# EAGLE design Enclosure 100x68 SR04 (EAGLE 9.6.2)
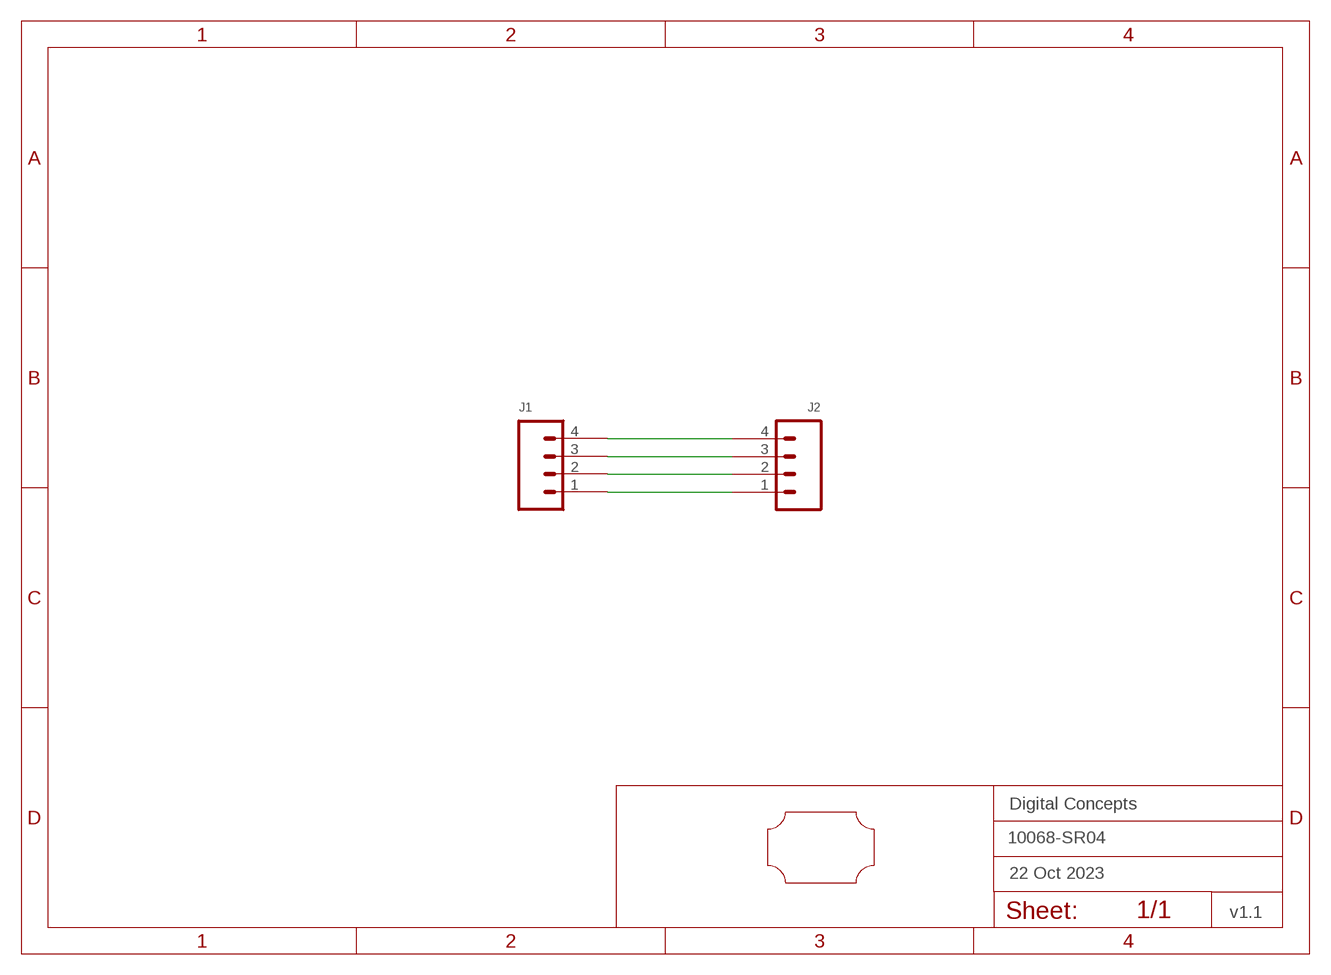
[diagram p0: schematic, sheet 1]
FRAME2 (FRAME_A5L-LOC): DATE: 22 Oct 2023; OWNER: Digital Concepts; TITLE: 10068-SR04; VERSION: v1.1

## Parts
J1  HEADER-1X4-GENERIC  [CONN_04-GENERIC]
J2  JST-XH2.54-4-HORIZONTAL  [JST-XH2.4-4-HORIZONTAL]
U$1  PROTO-34X22-SR04  [PROTO-34X22-SR04]

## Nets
N$1: J1.4 J2.4
N$2: J1.3 J2.3
N$3: J1.2 J2.2
N$4: J1.1 J2.1

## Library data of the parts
J1 = digitalconcepts:HEADER-1X4-GENERIC: Single Row 4-Pin Header
J2 = digitalconcepts:JST-XH2.54-4-HORIZONTAL: XH2.54 4P Horizontal Connector
U$1 = digitalconcepts:PROTO-34X22-SR04: 34 x 22 Prototyping board to fit an 100 x 68 enclosure—AJ-SR04M support

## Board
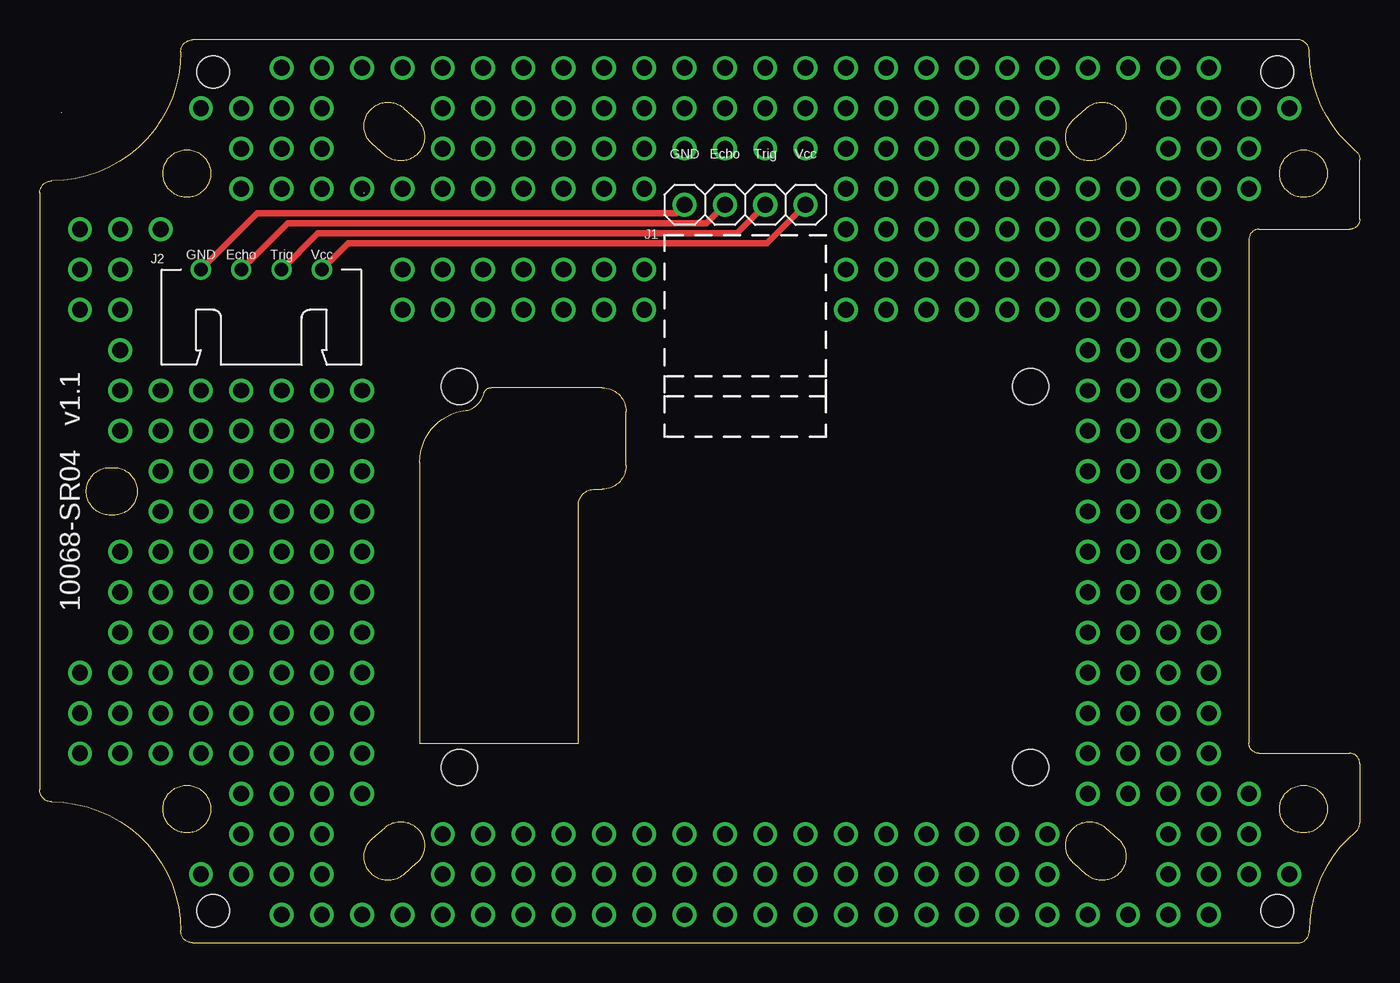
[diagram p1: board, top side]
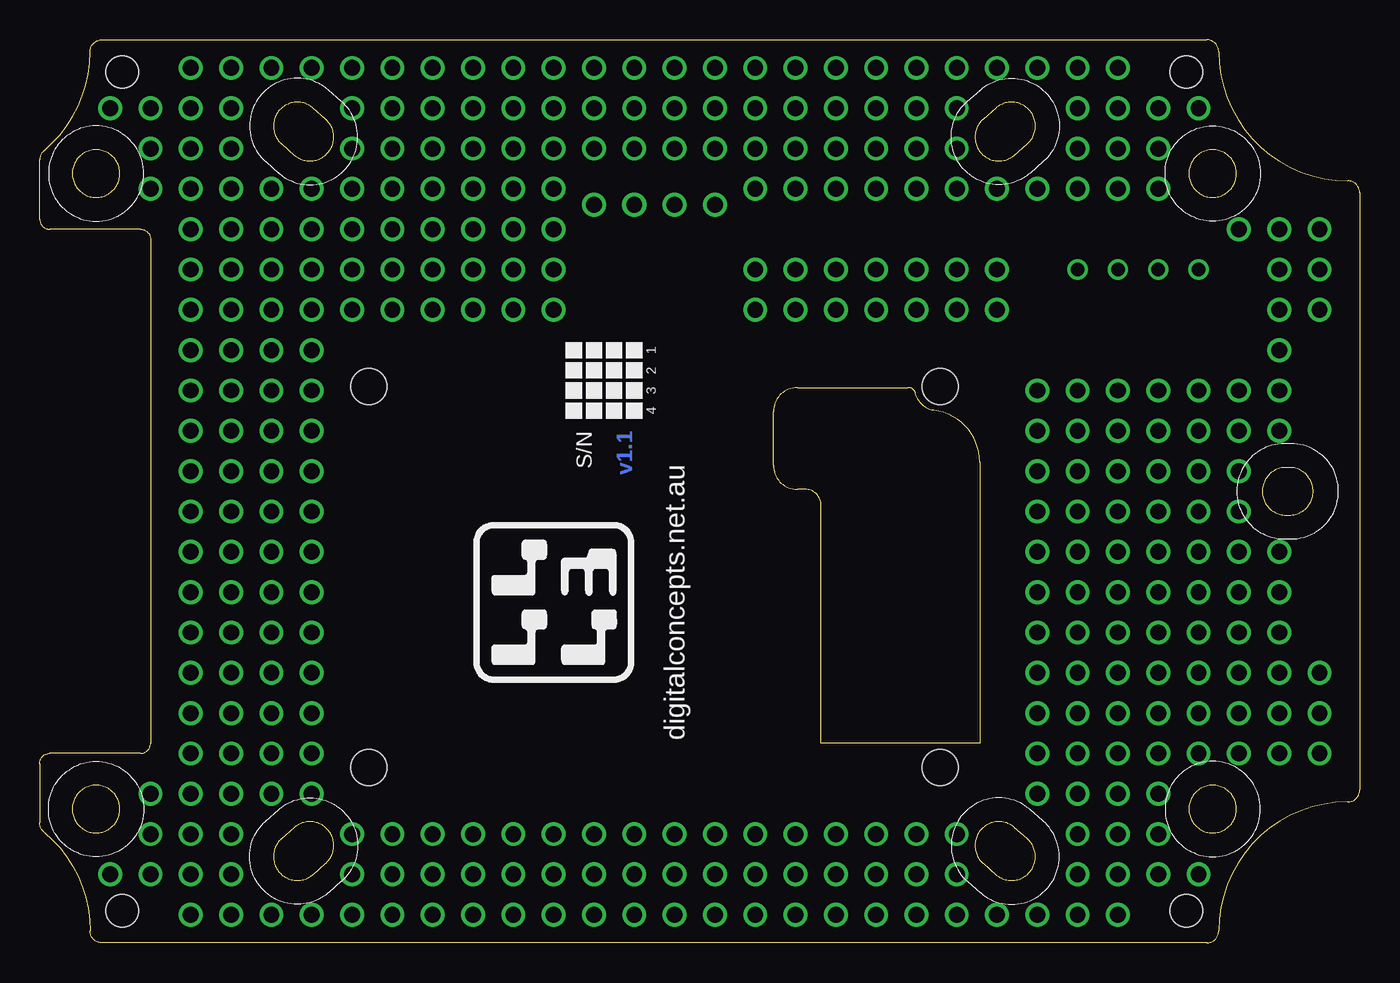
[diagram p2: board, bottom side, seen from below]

Size 83.19 x 56.9 mm. Coordinates in mm from the lower left corner, seen from the top.
Copper layers (1*16): Top 0.035mm / dielectric 1.5mm / Bottom 0.035mm
Design rules "default *": minimum track width 6mil, minimum drill 0.35mm, track to track 6mil, track to pad 6mil, pad to pad 6mil, via to via 6mil, smd to smd 6mil, copper to edge 6mil, drill to drill 6mil, minimum pad ring 1mil, minimum via ring 8mil, stop-mask expansion 4mil, vias tented up to drill 0mil, thermal gap 10mil

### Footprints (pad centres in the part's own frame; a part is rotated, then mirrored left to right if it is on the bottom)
CONN_04-GENERIC = drill 1 pad 1.524: 1 0,0; 2 2.54,0; 3 5.08,0; 4 7.62,0
JST-XH2.4-4-HORIZONTAL = drill 0.85: 1 3.81,0; 2 1.27,0; 3 -1.27,0; 4 -3.81,0
PROTO-34X22-SR04 = drill 1: P01-05 -41.91,-16.51; P01-06 -41.91,-13.97; P01-07 -41.91,-11.43; P01-16 -41.91,11.43; P01-17 -41.91,13.97; P01-18 -41.91,16.51; P02-05 -39.37,-16.51; P02-06 -39.37,-13.97; P02-07 -39.37,-11.43; P02-08 -39.37,-8.89; P02-09 -39.37,-6.35; P02-10 -39.37,-3.81; P02-13 -39.37,3.81; P02-14 -39.37,6.35; P02-15 -39.37,8.89; P02-16 -39.37,11.43; P02-17 -39.37,13.97; P02-18 -39.37,16.51; P03-05 -36.83,-16.51; P03-06 -36.83,-13.97; P03-07 -36.83,-11.43; P03-08 -36.83,-8.89; P03-09 -36.83,-6.35; P03-10 -36.83,-3.81; P03-11 -36.83,-1.27; P03-12 -36.83,1.27; P03-13 -36.83,3.81; P03-14 -36.83,6.35; P03-18 -36.83,16.51; P04-02 -34.29,-24.13; P04-05 -34.29,-16.51; P04-06 -34.29,-13.97; P04-07 -34.29,-11.43; P04-08 -34.29,-8.89; P04-09 -34.29,-6.35; P04-10 -34.29,-3.81; P04-11 -34.29,-1.27; P04-12 -34.29,1.27; P04-13 -34.29,3.81; P04-14 -34.29,6.35; P04-21 -34.29,24.13; P05-02 -31.75,-24.13; P05-03 -31.75,-21.59; P05-04 -31.75,-19.05; P05-05 -31.75,-16.51; P05-06 -31.75,-13.97; P05-07 -31.75,-11.43; P05-08 -31.75,-8.89; P05-09 -31.75,-6.35; P05-10 -31.75,-3.81; P05-11 -31.75,-1.27; P05-12 -31.75,1.27; P05-13 -31.75,3.81; P05-14 -31.75,6.35; P05-19 -31.75,19.05; P05-20 -31.75,21.59; P05-21 -31.75,24.13; P06-01 -29.21,-26.67; P06-02 -29.21,-24.13; P06-03 -29.21,-21.59; P06-04 -29.21,-19.05; P06-05 -29.21,-16.51; P06-06 -29.21,-13.97; P06-07 -29.21,-11.43; P06-08 -29.21,-8.89; P06-09 -29.21,-6.35; P06-10 -29.21,-3.81; P06-11 -29.21,-1.27; P06-12 -29.21,1.27; P06-13 -29.21,3.81; P06-14 -29.21,6.35; P06-19 -29.21,19.05; P06-20 -29.21,21.59; P06-21 -29.21,24.13; P06-22 -29.21,26.67; P07-01 -26.67,-26.67; P07-02 -26.67,-24.13; P07-03 -26.67,-21.59; P07-04 -26.67,-19.05; P07-05 -26.67,-16.51; P07-06 -26.67,-13.97; P07-07 -26.67,-11.43; P07-08 -26.67,-8.89; P07-09 -26.67,-6.35; P07-10 -26.67,-3.81; P07-11 -26.67,-1.27; P07-12 -26.67,1.27; P07-13 -26.67,3.81; P07-14 -26.67,6.35; P07-19 -26.67,19.05; P07-20 -26.67,21.59; P07-21 -26.67,24.13; P07-22 -26.67,26.67; P08-01 -24.13,-26.67; P08-04 -24.13,-19.05; P08-05 -24.13,-16.51; P08-06 -24.13,-13.97; P08-07 -24.13,-11.43; P08-08 -24.13,-8.89; P08-09 -24.13,-6.35; P08-10 -24.13,-3.81; P08-11 -24.13,-1.27; P08-12 -24.13,1.27; P08-13 -24.13,3.81; P08-14 -24.13,6.35; P08-19 -24.13,19.05; P08-22 -24.13,26.67; P09-01 -21.59,-26.67; P09-16 -21.59,11.43; P09-17 -21.59,13.97; P09-19 -21.59,19.05; P09-22 -21.59,26.67; P10-01 -19.05,-26.67; P10-02 -19.05,-24.13; P10-03 -19.05,-21.59; P10-16 -19.05,11.43; P10-17 -19.05,13.97; P10-19 -19.05,19.05; P10-20 -19.05,21.59; P10-21 -19.05,24.13; P10-22 -19.05,26.67; P11-01 -16.51,-26.67; P11-02 -16.51,-24.13; P11-03 -16.51,-21.59; P11-16 -16.51,11.43; P11-17 -16.51,13.97; P11-19 -16.51,19.05; P11-20 -16.51,21.59; P11-21 -16.51,24.13; P11-22 -16.51,26.67; P12-01 -13.97,-26.67; P12-02 -13.97,-24.13; P12-03 -13.97,-21.59; P12-16 -13.97,11.43; P12-17 -13.97,13.97; P12-19 -13.97,19.05; P12-20 -13.97,21.59; P12-21 -13.97,24.13; P12-22 -13.97,26.67; P13-01 -11.43,-26.67; P13-02 -11.43,-24.13; P13-03 -11.43,-21.59; P13-16 -11.43,11.43; P13-17 -11.43,13.97; P13-19 -11.43,19.05; P13-20 -11.43,21.59; P13-21 -11.43,24.13; P13-22 -11.43,26.67; P14-01 -8.89,-26.67; P14-02 -8.89,-24.13; P14-03 -8.89,-21.59; P14-16 -8.89,11.43; P14-17 -8.89,13.97; P14-19 -8.89,19.05; P14-20 -8.89,21.59; P14-21 -8.89,24.13; P14-22 -8.89,26.67; P15-01 -6.35,-26.67; P15-02 -6.35,-24.13; P15-03 -6.35,-21.59; P15-16 -6.35,11.43; P15-17 -6.35,13.97; P15-19 -6.35,19.05; P15-20 -6.35,21.59; P15-21 -6.35,24.13; P15-22 -6.35,26.67; P16-01 -3.81,-26.67; P16-02 -3.81,-24.13; P16-03 -3.81,-21.59; P16-20 -3.81,21.59; P16-21 -3.81,24.13; P16-22 -3.81,26.67; P17-01 -1.27,-26.67; P17-02 -1.27,-24.13; P17-03 -1.27,-21.59; P17-20 -1.27,21.59; P17-21 -1.27,24.13; P17-22 -1.27,26.67; P18-01 1.27,-26.67; P18-02 1.27,-24.13; P18-03 1.27,-21.59; P18-20 1.27,21.59; P18-21 1.27,24.13; P18-22 1.27,26.67; P19-01 3.81,-26.67; P19-02 3.81,-24.13; P19-03 3.81,-21.59; P19-20 3.81,21.59; P19-21 3.81,24.13; P19-22 3.81,26.67; P20-01 6.35,-26.67; P20-02 6.35,-24.13; P20-03 6.35,-21.59; P20-16 6.35,11.43; P20-17 6.35,13.97; P20-18 6.35,16.51; P20-19 6.35,19.05; P20-20 6.35,21.59; P20-21 6.35,24.13; P20-22 6.35,26.67; P21-01 8.89,-26.67; P21-02 8.89,-24.13; P21-03 8.89,-21.59; P21-16 8.89,11.43; P21-17 8.89,13.97; P21-18 8.89,16.51; P21-19 8.89,19.05; P21-20 8.89,21.59; P21-21 8.89,24.13; P21-22 8.89,26.67; P22-01 11.43,-26.67; P22-02 11.43,-24.13; P22-03 11.43,-21.59; P22-16 11.43,11.43; P22-17 11.43,13.97; P22-18 11.43,16.51; P22-19 11.43,19.05; P22-20 11.43,21.59; P22-21 11.43,24.13; P22-22 11.43,26.67; P23-01 13.97,-26.67; P23-02 13.97,-24.13; P23-03 13.97,-21.59; P23-16 13.97,11.43; P23-17 13.97,13.97; P23-18 13.97,16.51; P23-19 13.97,19.05; P23-20 13.97,21.59; P23-21 13.97,24.13; P23-22 13.97,26.67; P24-01 16.51,-26.67; P24-02 16.51,-24.13; P24-03 16.51,-21.59; P24-16 16.51,11.43; P24-17 16.51,13.97; P24-18 16.51,16.51; P24-19 16.51,19.05; P24-20 16.51,21.59; P24-21 16.51,24.13; P24-22 16.51,26.67; P25-01 19.05,-26.67; P25-02 19.05,-24.13; P25-03 19.05,-21.59; P25-16 19.05,11.43; P25-17 19.05,13.97; P25-18 19.05,16.51; P25-19 19.05,19.05; P25-20 19.05,21.59; P25-21 19.05,24.13; P25-22 19.05,26.67; P26-01 21.59,-26.67; P26-04 21.59,-19.05; P26-05 21.59,-16.51; P26-06 21.59,-13.97; P26-07 21.59,-11.43; P26-08 21.59,-8.89; P26-09 21.59,-6.35; P26-10 21.59,-3.81; P26-11 21.59,-1.27; P26-12 21.59,1.27; P26-13 21.59,3.81; P26-14 21.59,6.35; P26-15 21.59,8.89; P26-16 21.59,11.43; P26-17 21.59,13.97; P26-18 21.59,16.51; P26-19 21.59,19.05; P26-22 21.59,26.67; P27-01 24.13,-26.67; P27-04 24.13,-19.05; P27-05 24.13,-16.51; P27-06 24.13,-13.97; P27-07 24.13,-11.43; P27-08 24.13,-8.89; P27-09 24.13,-6.35; P27-10 24.13,-3.81; P27-11 24.13,-1.27; P27-12 24.13,1.27; P27-13 24.13,3.81; P27-14 24.13,6.35; P27-15 24.13,8.89; P27-16 24.13,11.43; P27-17 24.13,13.97; P27-18 24.13,16.51; P27-19 24.13,19.05; P27-22 24.13,26.67; P28-01 26.67,-26.67; P28-02 26.67,-24.13; P28-03 26.67,-21.59; P28-04 26.67,-19.05; P28-05 26.67,-16.51; P28-06 26.67,-13.97; P28-07 26.67,-11.43; P28-08 26.67,-8.89; P28-09 26.67,-6.35; P28-10 26.67,-3.81; P28-11 26.67,-1.27; P28-12 26.67,1.27; P28-13 26.67,3.81; P28-14 26.67,6.35; P28-15 26.67,8.89; P28-16 26.67,11.43; P28-17 26.67,13.97; P28-18 26.67,16.51; P28-19 26.67,19.05; P28-20 26.67,21.59; P28-21 26.67,24.13; P28-22 26.67,26.67; P29-01 29.21,-26.67; P29-02 29.21,-24.13; P29-03 29.21,-21.59; P29-04 29.21,-19.05; P29-05 29.21,-16.51; P29-06 29.21,-13.97; P29-07 29.21,-11.43; P29-08 29.21,-8.89; P29-09 29.21,-6.35; P29-10 29.21,-3.81; P29-11 29.21,-1.27; P29-12 29.21,1.27; P29-13 29.21,3.81; P29-14 29.21,6.35; P29-15 29.21,8.89; P29-16 29.21,11.43; P29-17 29.21,13.97; P29-18 29.21,16.51; P29-19 29.21,19.05; P29-20 29.21,21.59; P29-21 29.21,24.13; P29-22 29.21,26.67; P30-02 31.75,-24.13; P30-03 31.75,-21.59; P30-04 31.75,-19.05; P30-19 31.75,19.05; P30-20 31.75,21.59; P30-21 31.75,24.13; P31-02 34.29,-24.13; P31-21 34.29,24.13 | hole 2.032: -33.528,26.416; 33.528,26.416; 33.528,-26.416; -33.528,-26.416 | hole 2.25: -18,6.6; -18,-17.4; 18,6.6; 18,-17.4

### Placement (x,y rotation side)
J1  40.64,46.5 0 top
J2  13.97,42.42 180 top
U$1  44.45,28.45 0 top

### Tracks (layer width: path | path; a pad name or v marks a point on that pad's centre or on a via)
$X0
  cutout Bottom: 10.92,56.9 arc180 10.92,52.83 arc180
$X1
  cutout Bottom: 77.98,56.9 arc180 77.98,52.83 arc180
$X2
  cutout Bottom: 77.98,4.06 arc180 77.98,0 arc180
$X3
  cutout Bottom: 10.92,4.06 arc180 10.92,0 arc180
$X4
  cutout Top: 10.92,56.9 arc180 10.92,52.83 arc180
$X5
  cutout Top: 77.98,56.9 arc180 77.98,52.83 arc180
$X6
  cutout Top: 77.98,4.06 arc180 77.98,0 arc180
$X7
  cutout Top: 10.92,4.06 arc180 10.92,0 arc180
N$1
  Top 0.406: J2.4 19.43,44.07 45.83,44.07 J1.4
N$2
  Top 0.406: J2.3 17.53,44.7 43.93,44.7 J1.3
N$3
  Top 0.406: J2.2 15.62,45.34 42.02,45.34 J1.2
N$4
  Top 0.406: J2.1 13.72,45.97 40.12,45.97 J1.1

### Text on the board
Bottom: v1.1
tPlace: 10068-SR04 v1.1
bPlace: 1 | 2 | 3 | 4 | S/N | digitalconcepts.net.au
tNames: GND | Echo | Trig | Vcc | GND | Echo | Trig | Vcc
